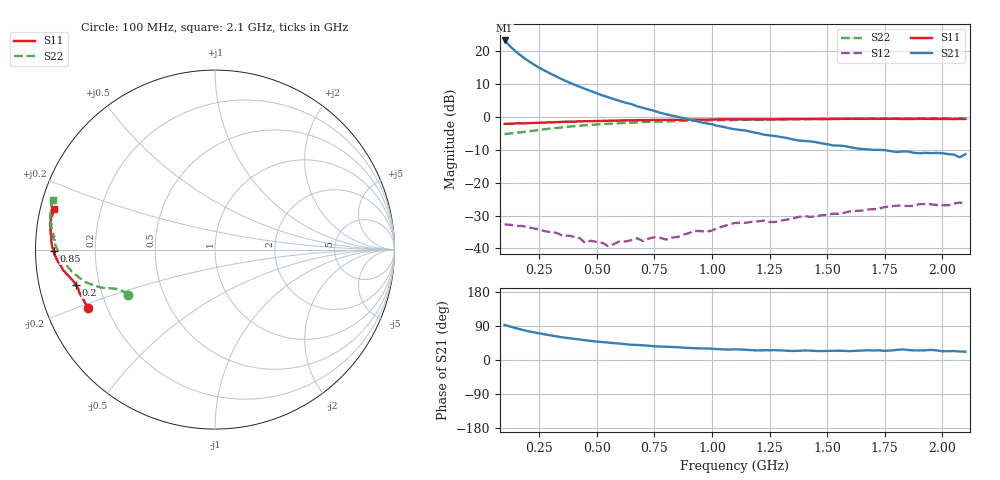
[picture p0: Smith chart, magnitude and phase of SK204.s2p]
!  POLYFET RF DEVICES
!  S PARAMETERS FOR
!  SK204 (EACH SIDE)
!  VDS=28, IDQ=800MA
! Date: Thu Sep 24 15:21:25 1998
! S2A 4Die, AP pkg, Vds=28Vdc, Idq=800ma, Vgsth=3.48Vdc
# MHZ  S  MA  R  50.0000
! SCATTERING PARAMETERS :
! Freq=MHz Mag[s11] Ang[s11] Mag[s21] Ang[s21] Mag[s12] Ang[s12] Mag[s22] Ang[s22]
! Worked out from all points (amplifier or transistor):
!   81 points, 100 MHz to 2.1 GHz, reference 50 ohm
!   highest |S21| = 23.2 dB at 100 MHz (marker M1)
!   |S21| within 3 dB of that: start of sweep to 142.9 MHz
!   unconditionally stable (mu >= 1): 400.1 MHz to end of sweep
!   at 425 MHz: K = 1.10, MAG = 21.1 dB, |S12| = -36.8 dB
!   at 1.1 GHz: K = 1.40, MAG = 10.5 dB, |S12| = -32.2 dB
!   at 2.1 GHz: K = 1.25, MAG = 4.5 dB, |S12| = -26.3 dB
!   S11 on the Smith chart (normalised r, x): 100 MHz: 0.13, -0.22; 200 MHz: 0.11, -0.12; 850 MHz: 0.05, -0.00; 2.1 GHz: 0.04, +0.12
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100  0.7797 -155.2  14.41 92.6  0.02319 6.3  0.5461 -152.4
125  0.7843 -159.1  11.64 88.1  0.02295 2.3  0.5585 -155.1
150  0.7922 -162.0  9.682 83.8  0.02203 1.1  0.5706 -156.7
175  0.7926 -164.0  8.285 79.9  0.02194 -1.1  0.5837 -157.7
200  0.8003 -165.7  7.153 76.3  0.02105 -2.4  0.598 -158.7
225  0.8056 -166.8  6.287 73.3  0.02017 -2.4  0.6133 -159.3
250  0.8107 -167.8  5.555 70.4  0.01952 -1.3  0.63 -160.1
300  0.8225 -169.1  4.51 64.9  0.01773 -2.8  0.6622 -161.3
350  0.8361 -170.5  3.691 59.7  0.01577 -4.0  0.6889 -162.8
400  0.8443 -171.6  3.103 56.0  0.0151 2.2  0.7194 -164.5
450  0.8563 -172.6  2.643 51.9  0.01208 8.5  0.7451 -166.0
525  0.8658 -174.3  2.111 47.3  0.01214 20.4  0.7744 -168.5
575  0.8725 -175.1  1.852 44.5  0.01166 31.7  0.7912 -169.8
675  0.8871 -176.8  1.44 39.8  0.01428 44.5  0.8223 -172.9
700  0.8879 -177.2  1.369 38.8  0.01298 45.6  0.8323 -174.0
775  0.8934 -178.3  1.151 35.6  0.01454 53.4  0.8442 -175.4
850  0.8974 -179.6  1 33.7  0.01492 63.7  0.8621 -177.3
1100  0.9138 176.9  0.6449 28.0  0.02442 78.7  0.8916 177.0
1450  0.9227 173.1  0.4122 23.8  0.03073 87.4  0.9214 171.2
1775  0.9323 168.8  0.3015 24.9  0.04347 87.8  0.938 166.6
2075  0.926 166.1  0.2423 22.3  0.04994 87.1  0.946 163.3
2100  0.9262 166.0  0.2702 21.9  0.04822 84.9  0.9437 162.9
